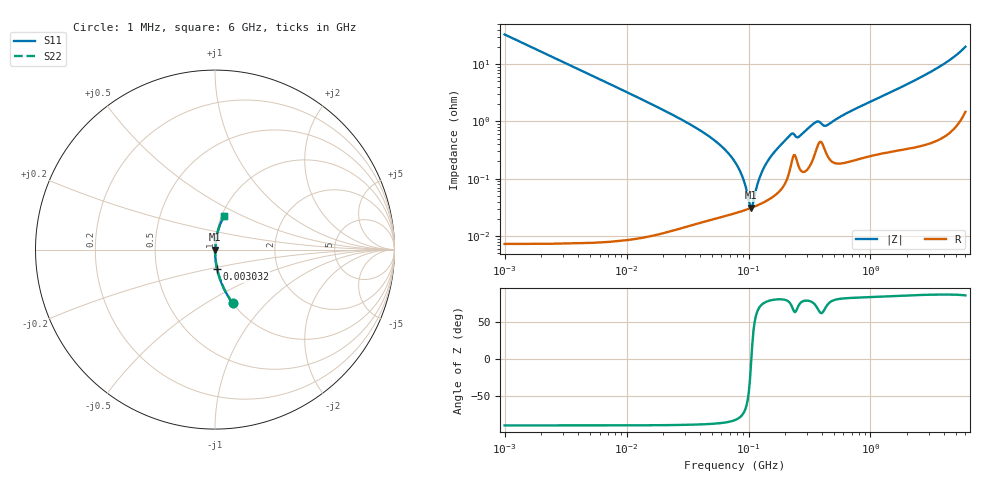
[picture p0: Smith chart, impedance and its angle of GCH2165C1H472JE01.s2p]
!Murata Part Number: GCH2165C1H472JE01
!These Parameters are Measured in Series Mode Connection
!Data Generated on Jun 19, 2026
!  o--ll--o
!Port1  Port2
!  o------o
!Operation Temp=25[degC], DC Bias Voltage=0[V]
!Freq. Start=1000[kHz] Stop=6[GHz] 401[Steps]
# Hz S RI R 50
!Freq.(Hz) S11(Real) S11(Imag) S21(Real) S21(Imag) S12(Real) S12(Imag) S22(Real) S22(Imag)
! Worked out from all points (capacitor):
!   401 points, 1 MHz to 6 GHz, reference 50 ohm
!   read as one part in series: C = 4.84 nF near 1.044 MHz
!   lowest |Z| = 31.1 mohm at 105 MHz (marker M1)
!   series resonance near 105.5 MHz, so ESL is about 470 pH
!   S11 on the Smith chart (normalised r, x): 1 MHz: 1.00, -0.66; 3.032 MHz: 1.00, -0.22; 6 GHz: 1.03, +0.40
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1000000  0.0977 -0.2969  0.9023 0.2969  0.9023 0.2969  0.0977 -0.2969
3031896  0.0117 -0.1072  0.9883 0.1072  0.9883 0.1072  0.0117 -0.1072
4293785  0.00589 -0.076  0.9941 0.076  0.9941 0.076  0.00589 -0.076
1.843659e7  0.000405 -0.0172  0.9996 0.0172  0.9996 0.0172  0.000405 -0.0172
4.800399e7  0.000218 -0.00539  0.9998 0.00539  0.9998 0.00539  0.000218 -0.00539
6.368941e7  0.000232 -0.00326  0.9998 0.00326  0.9998 0.00326  0.000232 -0.00326
7.745967e7  0.000253 -0.00194  0.9997 0.00194  0.9997 0.00194  0.000253 -0.00194
8.825674e7  0.000273 -0.00111  0.9997 0.00111  0.9997 0.00111  0.000273 -0.00111
1.005588e8  0.000299 -0.000296  0.9997 0.000296  0.9997 0.000296  0.000299 -0.000296
1.050294e8  0.00031 -2.5e-05  0.9997 2.5e-05  0.9997 2.5e-05  0.00031 -2.5e-05
1.096987e8  0.000321 0.000246  0.9997 -0.000246  0.9997 -0.000246  0.000321 0.000246
1.196694e8  0.000348 0.000794  0.9997 -0.000794  0.9997 -0.000794  0.000348 0.000794
1.277378e8  0.000372 0.00121  0.9996 -0.00121  0.9996 -0.00121  0.000372 0.00121
1.553559e8  0.000475 0.00253  0.9995 -0.00253  0.9995 -0.00253  0.000475 0.00253
2.200158e8  0.00156 0.00562  0.9984 -0.00562  0.9984 -0.00562  0.00156 0.00562
2.561955e8  0.00172 0.00503  0.9983 -0.00503  0.9983 -0.00503  0.00172 0.00503
3.325952e8  0.00209 0.00847  0.9979 -0.00847  0.9979 -0.00847  0.00209 0.00847
3.708027e8  0.00394 0.00916  0.9961 -0.00916  0.9961 -0.00916  0.00394 0.00916
4.412715e8  0.00263 0.00817  0.9974 -0.00817  0.9974 -0.00817  0.00263 0.00817
1.428092e9  0.00388 0.0312  0.9961 -0.0312  0.9961 -0.0312  0.00388 0.0312
3.483508e9  0.0115 0.0826  0.9885 -0.0826  0.9885 -0.0826  0.0115 0.0826
6e9  0.0514 0.1873  0.9486 -0.1873  0.9486 -0.1873  0.0514 0.1873
